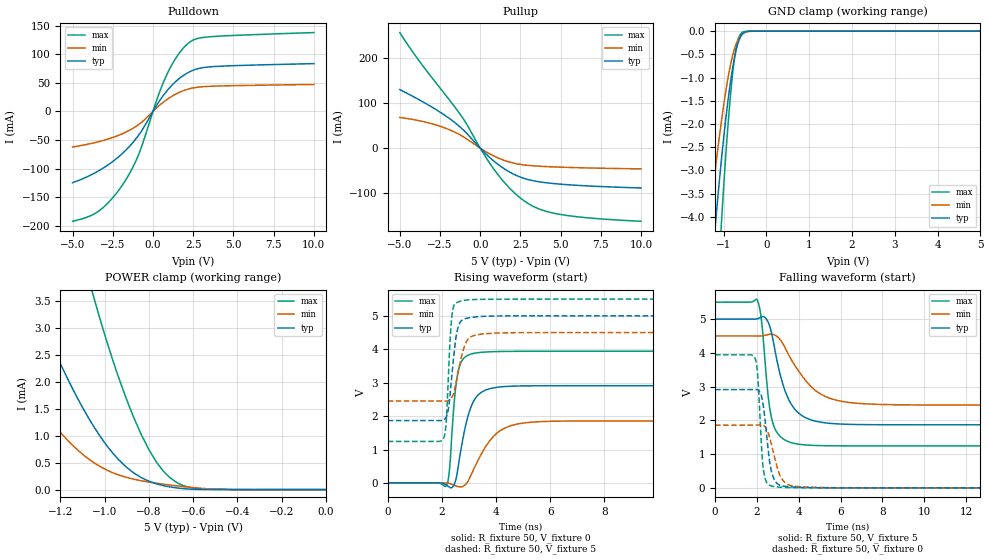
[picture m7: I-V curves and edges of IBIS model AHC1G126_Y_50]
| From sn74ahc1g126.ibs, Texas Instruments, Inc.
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[Model]   AHC1G126_Y_50
Model_type  3-state
Enable   Active-High
Vref =   0
Rref =   1000
Cref =   50p
Vmeas =   2.5
| variable   typ   min   max
C_comp   2.66pF   2.26pF   2.87pF
| C_pullup   3.93pF   2.48pF   5.16pF
| C_pulldown   4.88pF   2.72pF   8.61pF
| C_tri-state   2.66pF   2.26pF   2.87pF
[Temperature Range]   40   100   -40
| Ambient temperature   25   85   -40
[Voltage range]   5   4.5   5.5
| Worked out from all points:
|   slope of the pulldown table from 0 to 0.75 V, typ, clamps not added: 23.5 ohm
|   slope of the pullup table from 0 to 0.75 V, typ, clamps not added: 29 ohm
|   GND clamp passes 1 mA (typ) near -0.82 V on its own axis
|   POWER clamp passes 1 mA (typ) near -1.02 V on its own axis
|   rising waveform, R_fixture 50, V_fixture 0: 20-80 % time 481ps typ, 874ps min, 241ps max; typ from 0 V to 2.91 V
|   falling waveform, R_fixture 50, V_fixture 5: 20-80 % time 853ps typ, 1.45ns min, 422ps max; typ from 5 V to 1.87 V
|   rising waveform, R_fixture 50, V_fixture 5: 20-80 % time 241ps typ, 344ps min, 152ps max; typ from 1.87 V to 5 V
|   falling waveform, R_fixture 50, V_fixture 0: 20-80 % time 333ps typ, 491ps min, 212ps max; typ from 2.91 V to 0 V
[GND Clamp]
| AHC1G126_Y_50
|   Voltage   I(typ)   I(min)   I(max)
-5V       -82.2mA    -53.18mA   -120.1mA
-1.345V   -5.939mA   -4.23mA    -9.455mA
-1.325V   -5.698mA   -4.059mA   -9.052mA
-1.18V    -4.064mA   -2.884mA   -6.306mA
-1.08V    -3.056mA   -2.15mA    -4.612mA
-1.045V   -2.728mA   -1.909mA   -4.063mA
-900mV    -1.524mA   -1.032mA   -2.071mA
-825mV    -1.015mA   -673.6uA   -1.254mA
-760mV    -650.5uA   -429.5uA   -694.5uA
-660mV    -253.8uA   -181.4uA   -175.8uA
-540mV    -43.74uA   -45.9uA    -14.62uA
5V        202.2pA    7.882uA    5.191pA
[POWER Clamp]
| AHC1G126_Y_50
|   Voltage   I(typ)   I(min)   I(max)
-5V       84.23mA    53.81mA    136.8mA
-1.595V   6.677mA    3.573mA    14.16mA
-1.34V    3.677mA    1.806mA    8.607mA
-1.19V    2.243mA    1.013mA    5.808mA
-1.07V    1.306mA    558.7uA    3.866mA
-1.045V   1.14mA     487.9uA    3.498mA
-940mV    566.9uA    276.1uA    2.112mA
-835mV    223.3uA    164.8uA    1.022mA
-765mV    105.5uA    117.7uA    503.4uA
-705mV    49.45uA    84.73uA    220uA
-580mV    3.937uA    29.62uA    18.37uA
-84.45fV  202.2pA    739.6pA    6.479pA
[Pulldown]
| AHC1G126_Y_50
|   Voltage   I(typ)   I(min)   I(max)
-5V       -124.7mA   -62.26mA   -192.3mA
-3.32V    -103mA     -52.53mA   -173.4mA
-2.555V   -88.79mA   -46.08mA   -152.8mA
-1.805V   -71.05mA   -37.71mA   -124.9mA
-860mV    -40.28mA   -22.34mA   -73.34mA
270mV     12.63mA    7.355mA    23.03mA
845mV     35.27mA    20.53mA    63.42mA
1.525V    55.18mA    31.97mA    97.85mA
2.23V     68.77mA    39.46mA    120.3mA
2.725V    74.39mA    42.27mA    127.4mA
3.55V     78.14mA    44.07mA    130.9mA
10V       83.81mA    47.29mA    138.2mA
[Pullup]
| AHC1G126_Y_50
|   Voltage   I(typ)   I(min)   I(max)
-5V       130.5mA    68.31mA    257.4mA
-3.72V    106.1mA    60.5mA     190.6mA
-1.735V   61.15mA    38.13mA    98.98mA
-925mV    36.03mA    22.44mA    58.1mA
130mV     -4.903mA   -3.064mA   -7.764mA
895mV     -30.26mA   -18.39mA   -49.05mA
1.71V     -50.82mA   -29.82mA   -84.75mA
2.525V    -64.92mA   -36.51mA   -111.9mA
3.53V     -74.18mA   -39.96mA   -133.6mA
4.765V    -79.55mA   -42.12mA   -146.3mA
6.775V    -84.33mA   -44.19mA   -155.5mA
10V       -88.72mA   -46.22mA   -163mA
[Ramp]
| AHC1G126_Y_50
| variable   typ   min   max
dV/dt_r   1.83/4.93E-10   1.18/8.96E-10   2.43/2.49E-10
dV/dt_f   1.92/8.60E-10   1.26/1.46E-09   2.61/4.32E-10
R_load = 50
[Rising Waveform]
| AHC1G126_Y_50
R_fixture =   50
C_fixture =   0
L_fixture =   0
V_fixture =   0
V_fixture_min = 0
V_fixture_max = 0
|   Time   V(typ)   V(min)   V(max)
0s        163.8pV    254.3pV    77.37pV
2.165ns   -63.99mV   -1.488mV   -90.62mV
2.275ns   -122.7mV   -17.82mV   362.5mV
2.455ns   -42.61mV   -67.73mV   2.413V
2.6ns     478.4mV    -108.6mV   3.336V
2.905ns   1.817V     -16.56mV   3.796V
3.195ns   2.48V      446.4mV    3.88V
4.06ns    2.865V     1.508V     3.932V
5.315ns   2.906V     1.819V     3.94V
24.99ns   2.91V      1.856V     3.94V
[Falling Waveform]
| AHC1G126_Y_50
R_fixture =   50
C_fixture =   0
L_fixture =   0
V_fixture =   5
V_fixture_min = 4.5
V_fixture_max = 5.5
|   Time   V(typ)   V(min)   V(max)
0s        5V         4.5V       5.5V
2.02ns    5.009V     4.499V     5.564V
2.21ns    5.057V     4.5V       5.018V
2.53ns    4.919V     4.539V     2.773V
2.72ns    4.54V      4.55V      2.024V
3.19ns    3.182V     4.322V     1.482V
3.68ns    2.443V     3.762V     1.333V
4.925ns   1.959V     2.826V     1.253V
6.63ns    1.878V     2.514V     1.243V
24.99ns   1.868V     2.452V     1.242V
[Rising Waveform]
| AHC1G126_Y_50
R_fixture =   50
C_fixture =   0
L_fixture =   0
V_fixture =   5
V_fixture_min = 4.5
V_fixture_max = 5.5
|   Time   V(typ)   V(min)   V(max)
0s        1.868V     2.452V     1.242V
2.055ns   1.883V     2.45V      1.321V
2.155ns   1.969V     2.45V      1.771V
2.31ns    2.712V     2.493V     4.376V
2.39ns    3.395V     2.595V     5.112V
2.555ns   4.514V     3.119V     5.401V
2.775ns   4.889V     3.938V     5.455V
3.1ns     4.951V     4.386V     5.485V
4.155ns   4.997V     4.489V     5.498V
24.99ns   5V         4.5V       5.5V
[Falling Waveform]
| AHC1G126_Y_50
R_fixture =   50
C_fixture =   0
L_fixture =   0
V_fixture =   0
V_fixture_min = 0
V_fixture_max = 0
|   Time   V(typ)   V(min)   V(max)
0s        2.91V      1.856V     3.94V
1.92ns    2.915V     1.858V     3.827V
2.045ns   2.899V     1.862V     3.278V
2.225ns   2.706V     1.867V     1.221V
2.31ns    2.421V     1.853V     549.7mV
2.46ns    1.609V     1.744V     171.4mV
2.72ns    432.8mV    1.227V     50.15mV
3.2ns     61.11mV    263.8mV    16.58mV
3.965ns   16.54mV    38.07mV    4.011mV
24.99ns   163.9pV    4.489nV    77.27pV
